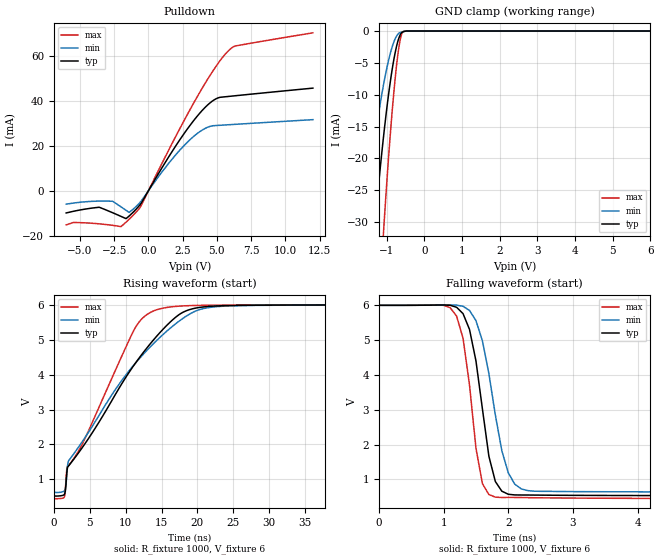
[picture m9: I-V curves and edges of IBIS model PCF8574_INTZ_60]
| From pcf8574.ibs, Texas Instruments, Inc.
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[Model]   PCF8574_INTZ_60
Model_type  Open_drain
Enable   Active-Low
Vref =   6.0
Rref =   4700
Cref =   10p
Vmeas =   3.0
| variable   typ   min   max
C_comp   0.76pF   0.70pF   0.88pF
| C_pulldown   0.72pF   0.67pF   0.79pF
| C_tri-state   0.76pF   0.70pF   0.88pF
[Temperature Range]   40   100   -40
| Ambient temperature   25   85   -40
[Voltage range]   6   6   6
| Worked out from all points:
|   slope of the pulldown table from 0 to 0.9 V, typ, clamps not added: 96.4 ohm
|   GND clamp passes 1 mA (typ) near -0.67 V on its own axis
|   rising waveform, R_fixture 1000, V_fixture 6: 20-80 % time 10.6ns typ, 11.4ns min, 7.62ns max; typ from 0.523 V to 6 V
|   falling waveform, R_fixture 1000, V_fixture 6: 20-80 % time 262ps typ, 314ps min, 221ps max; typ from 6 V to 0.523 V
[GND Clamp]
| PCF8574_INTZ_60
|   Voltage   I(typ)   I(min)   I(max)
-6V       -503mA     -362.9mA   -755.6mA
-1.59V    -50.07mA   -31.23mA   -86.94mA
-1.315V   -30.65mA   -17.09mA   -55.3mA
-1.09V    -17.08mA   -8.725mA   -32.39mA
-1.07V    -16mA      -8.086mA   -30.53mA
-955mV    -10.3mA    -4.8mA     -20.48mA
-835mV    -5.423mA   -2.19mA    -11.44mA
-740mV    -2.521mA   -841.1uA   -5.637mA
-655mV    -817.5uA   -281uA     -1.891mA
-580mV    -176.9uA   -129.9uA   -212.1uA
-480mV    -4.521uA   -8.928uA   -1.527uA
6V        503.8pA    636.2pA    144.6pA
[Pulldown]
| PCF8574_INTZ_60
|   Voltage   I(typ)   I(min)   I(max)
-6V       -9.886mA   -5.97mA    -15.23mA
-3.59V    -7.335mA   -4.599mA   -14.73mA
-2.615V   -9.767mA   -4.664mA   -15.39mA
-2.01V    -11.38mA   -7.122mA   -15.96mA
-1.41V    -11.26mA   -9.634mA   -12.71mA
-970mV    -8.676mA   -7.415mA   -9.978mA
-525mV    -5.514mA   -4.568mA   -6.543mA
1.605V    16.31mA    13.18mA    19.64mA
3.28V     31.11mA    24.12mA    38.86mA
4.76V     40.38mA    29.03mA    53.92mA
6.045V    42.18mA    29.51mA    63.54mA
12V       45.76mA    31.71mA    70.42mA
[Ramp]
| PCF8574_INTZ_60
| variable   typ   min   max
dV/dt_r   3.29/1.06E-08   3.23/1.14E-08   3.33/7.61E-09
dV/dt_f   3.29/2.59E-10   3.23/3.13E-10   3.34/2.13E-10
R_load = 1000
[Rising Waveform]
| PCF8574_INTZ_60
R_fixture =   1000
C_fixture =   0
L_fixture =   0
V_fixture =   6
V_fixture_min = 6
V_fixture_max = 6
|   Time   V(typ)   V(min)   V(max)
0s        522.6mV    626mV      446.4mV
1.5ns     579.7mV    678.3mV    512.6mV
1.7ns     888.6mV    839.5mV    1.012V
1.9ns     1.341V     1.375V     1.367V
4.1ns     1.952V     2.123V     2.069V
11.5ns    4.37V      4.363V     5.398V
16.6ns    5.582V     5.399V     5.95V
20.7ns    5.939V     5.888V     5.989V
28ns      5.991V     5.986V     5.998V
269.9ns   6V         6V         6V
[Falling Waveform]
| PCF8574_INTZ_60
R_fixture =   1000
C_fixture =   0
L_fixture =   0
V_fixture =   6
V_fixture_min = 6
V_fixture_max = 6
|   Time   V(typ)   V(min)   V(max)
0s        6V         6V         6V
1.1ns     6.001V     6.011V     5.931V
1.3ns     5.761V     5.971V     5.054V
1.5ns     4.402V     5.559V     1.895V
1.6ns     3.021V     4.979V     876.7mV
1.7ns     1.664V     4.036V     566.2mV
1.9ns     662.2mV    1.826V     481.2mV
2.2ns     552.5mV    728.5mV    479.6mV
3.8ns     537.9mV    644.7mV    457mV
269.9ns   522.6mV    626mV      446.4mV
